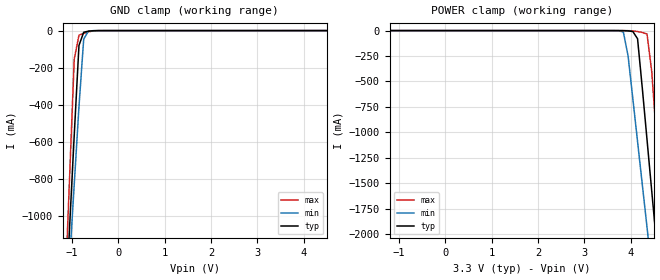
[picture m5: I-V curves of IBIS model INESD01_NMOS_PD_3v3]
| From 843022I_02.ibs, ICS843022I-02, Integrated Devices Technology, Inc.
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[Model] INESD01_NMOS_PD_3v3
Model_type   Input
Polarity   Non-Inverting
Vinl = 0.7V
Vinh = 1.3V
|   typ   min   max
C_comp   2pF   1.5pF   2.5pF
|   typ   min   max
[Voltage range]  3.3V   3.15V   3.45V
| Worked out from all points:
|   GND clamp passes 1 mA (typ) near -0.56 V on its own axis
[GND_clamp]
|Voltage   I(typ)   I(min)   I(max)
-3.3V     -12.24A    -10.56A    -15.06A
-1.157V   -1.578A    -1.673A    -1.45A
-1.055V   -1.071A    -1.251A    -801.8mA
-952.6mV  -564.4mA   -830.8mA   -154mA
-850.5mV  -79.94mA   -410.9mA   -24.98mA
-748.5mV  -8.971mA   -45.88mA   -14.67mA
-646.4mV  -3.031mA   -2.844mA   -6.635mA
-544.3mV  -662.6uA   -322.8uA   -1.644mA
6.6V      128uA      160uA      99.15uA
[POWER_clamp]
|Voltage   I(typ)   I(min)   I(max)
-3.3V     128uA      156uA      101.6uA
3.64V     -11.65uA   -147.3uA   -2.645uA
3.844V    -662.6uA   -14.52mA   -37.72uA
3.946V    -3.031mA   -250.2mA   -458.6uA
4.048V    -8.971mA   -669.7mA   -3.092mA
4.151V    -79.94mA   -1.09A     -9.452mA
4.355V    -1.071A    -1.933A    -33.36mA
4.457V    -1.578A    -2.355A    -402.2mA
4.559V    -2.085A    -2.777A    -1.05A
4.661V    -2.593A    -3.199A    -1.698A
4.763V    -3.101A    -3.622A    -2.347A
6.6V      -12.24A    -11.24A    -14.01A
